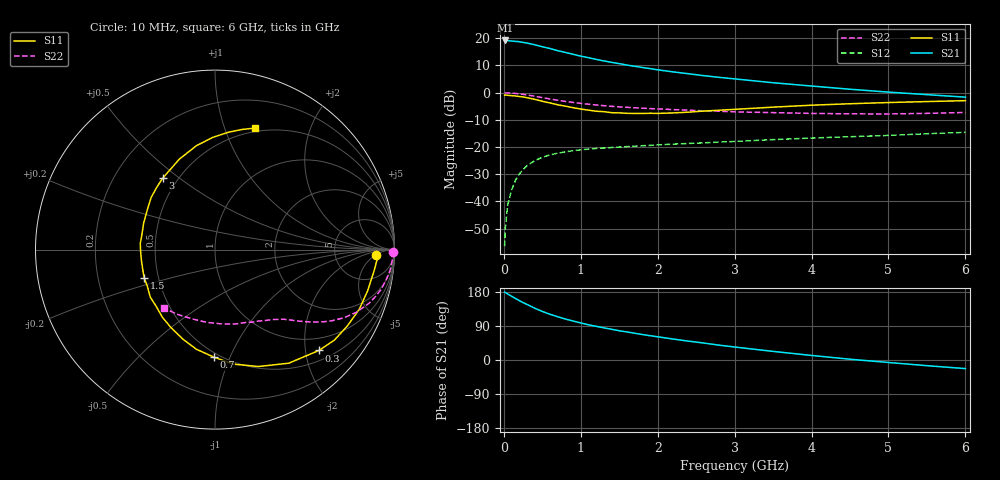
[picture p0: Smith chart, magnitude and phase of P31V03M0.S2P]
! SIEMENS Small Signal Semiconductors
! BFP181
! Si NPN RF Bipolar Junction Transistor in SOT143
! VCE = 1 V  IC = 3 mA
! Common Emitter S-Parameters:  March  1996
# GHz  S  MA  R  50
!  f  S11  S21  S12  S22
! GHz  MAG  ANG  MAG  ANG  MAG  ANG  MAG  ANG
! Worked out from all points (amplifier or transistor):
!   36 points, 10 MHz to 6 GHz, reference 50 ohm
!   highest |S21| = 19.2 dB at 20 MHz (marker M1)
!   |S21| within 3 dB of that: start of sweep to 604 MHz
!   unconditionally stable (mu >= 1): 1.901 GHz to end of sweep
!   at 250 MHz: K = 0.17, MSG = 23.4 dB, |S12| = -28.3 dB
!   at 1.4 GHz: K = 0.82, MSG = 15.7 dB, |S12| = -20.2 dB
!   at 6 GHz: K = 1.16, MAG = 4.1 dB, |S12| = -14.6 dB
!   S11 on the Smith chart (normalised r, x): 10 MHz: 17, -5; 300 MHz: 0.71, -2.28; 700 MHz: 0.47, -0.87; 1.5 GHz: 0.42, -0.16; 3 GHz: 0.41, +0.44; 6 GHz: 0.46, +1.28
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0.01  0.8981 -1.8  9.108 179.1  0.0015 87.1  0.9924 -0.7
0.02  0.9058 -3.2  9.134 178.2  0.0033 88.6  0.9864 -1.3
0.05  0.8948 -7.4  9.069 174.2  0.0086 88.2  0.9893 -3.5
0.1  0.8807 -15.2  8.921 168.3  0.016 80.7  0.9818 -6.9
0.2  0.851 -30.1  8.665 156.9  0.0317 72.9  0.9521 -13.4
0.25  0.8347 -37.2  8.42 151.4  0.0384 69.3  0.9309 -16.4
0.3  0.8071 -44.1  8.202 146.8  0.0453 65.6  0.909 -19.2
0.4  0.7546 -57.0  7.615 136.7  0.056 58.8  0.8609 -24.0
0.5  0.695 -69.6  7.002 128.1  0.0647 52.9  0.8121 -27.9
0.6  0.6465 -80.8  6.49 120.7  0.0717 48.3  0.7658 -31.1
0.7  0.5988 -90.7  5.919 114.2  0.077 44.8  0.7252 -33.7
0.9  0.5304 -109.6  5.082 102.9  0.0857 39.1  0.6615 -37.5
1.1  0.4775 -127.9  4.402 92.9  0.0918 35.2  0.613 -40.5
1.3  0.4473 -143.7  3.836 84.9  0.0959 32.2  0.5763 -42.9
1.5  0.4249 -158.4  3.418 77.2  0.0999 30.5  0.5478 -45.1
1.8  0.4147 -178.7  2.907 67.2  0.1057 28.5  0.5184 -48.6
2.2  0.424 159.6  2.411 55.3  0.113 26.3  0.4887 -53.7
3  0.4933 126.2  1.793 34.3  0.1267 23.1  0.4438 -65.7
3.5  0.5418 111.5  1.523 22.7  0.137 21.1  0.4295 -74.9
4.5  0.6258 91.0  1.157 2.1  0.1549 16.2  0.4081 -96.6
5.5  0.6862 77.3  0.92 -15.0  0.1757 12.1  0.4164 -119.5
6  0.7131 71.7  0.827 -22.7  0.1865 9.2  0.4324 -131.0
